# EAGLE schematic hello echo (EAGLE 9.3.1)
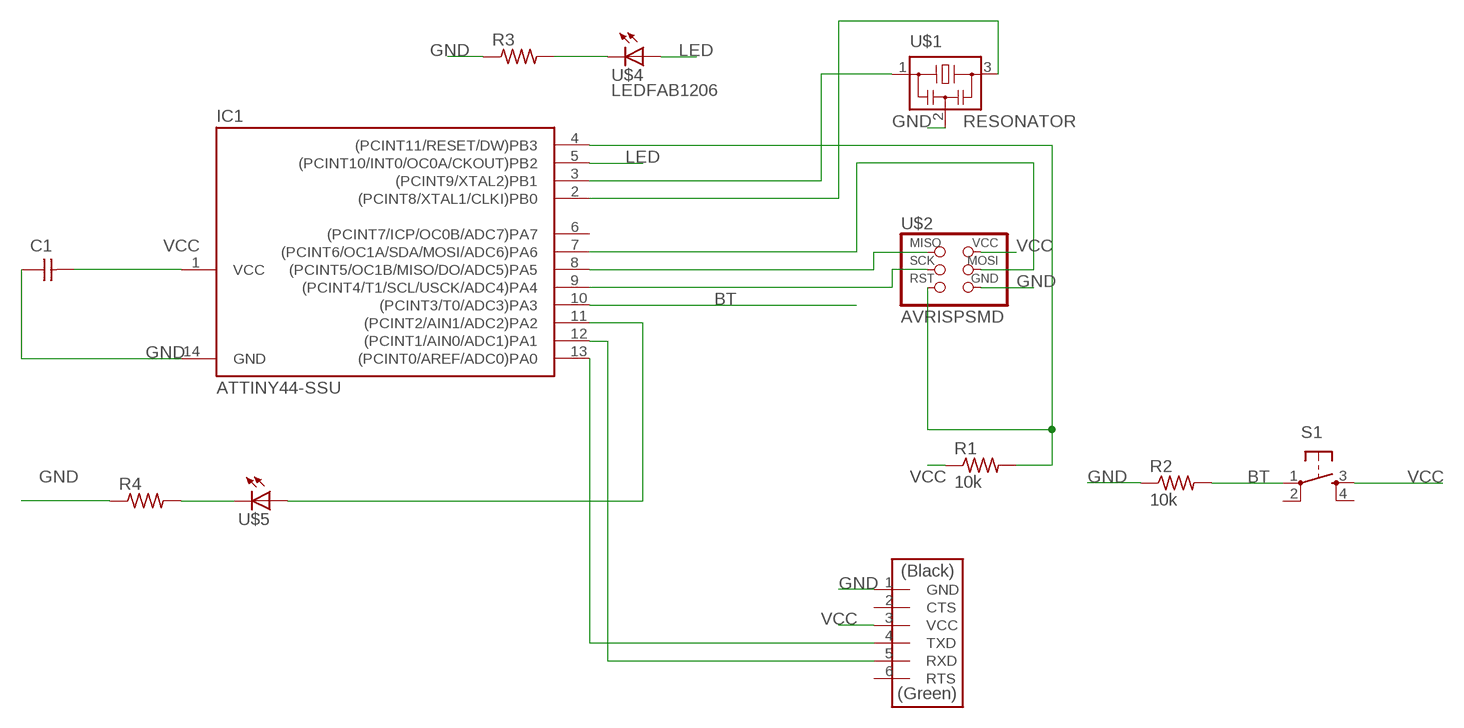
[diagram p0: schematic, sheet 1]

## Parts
C1  1uF  CAP-UNPOLARIZEDFAB  [C1206FAB]
IC1  ATTINY44-SSU  [SOIC14]
R1  10k  RES-US1206FAB  [R1206FAB]
R2  10k  RES-US1206FAB  [R1206FAB]
R3  RES-US1206FAB  [R1206FAB]
R4  RES-US1206FAB  [R1206FAB]
S1  6MM_SWITCH6MM_SWITCH  [6MM_SWITCH]
U$1  RESONATOR  [EFOBM]
U$2  AVRISPSMD  [2X03SMD]
U$3  FTDI-SMD-HEADER  [1X06SMD]
U$4  LEDFAB1206  [LED1206FAB]
U$5  LEDFAB1206  [LED1206FAB]

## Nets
BT: IC1.10((PCINT3/T0/ADC3)PA3) R2.2 S1.1(P)
GND: C1.1 IC1.14(GND) R2.1 R3.1 R4.1 U$1.2 U$2.6(GND) U$3.1(GND)
LED: IC1.5((PCINT10/INT0/OC0A/CKOUT)PB2) U$4.1(A)
N$1: R3.2 U$4.2(C)
N$2: R4.2 U$5.2(C)
N$3: IC1.3((PCINT9/XTAL2)PB1) U$1.1
N$4: IC1.2((PCINT8/XTAL1/CLKI)PB0) U$1.3
N$5: IC1.11((PCINT2/AIN1/ADC2)PA2) U$5.1(A)
N$7: IC1.4((PCINT11/RESET/DW)PB3) R1.2 U$2.5(RST)
N$8: IC1.7((PCINT6/OC1A/SDA/MOSI/ADC6)PA6) U$2.4(MOSI)
N$9: IC1.8((PCINT5/OC1B/MISO/DO/ADC5)PA5) U$2.1(MISO)
N$10: IC1.9((PCINT4/T1/SCL/USCK/ADC4)PA4) U$2.3(SCK)
N$13: IC1.13((PCINT0/AREF/ADC0)PA0) U$3.4(TXD)
N$14: IC1.12((PCINT1/AIN0/ADC1)PA1) U$3.5(RXD)
VCC: C1.2 IC1.1(VCC) R1.1 S1.3(S) U$2.2(VCC) U$3.3(VCC)
Unconnected: IC1.6((PCINT7/ICP/OC0B/ADC7)PA7) S1.2(P1) S1.4(S1) U$3.2(CTS) U$3.6(RTS)

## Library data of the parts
C1 = fab:CAP-UNPOLARIZED
IC1 = fab:ATTINY44
R1-R4 = fab:RES-US: Resistor (US Symbol)
S1 = fab:6MM_SWITCH: OMRON SWITCH
U$1 = fab:RESONATOR
U$2 = fab:AVRISP
U$3 = fab:FTDI-SMD-HEADER
U$4 U$5 = fab:LED: LED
